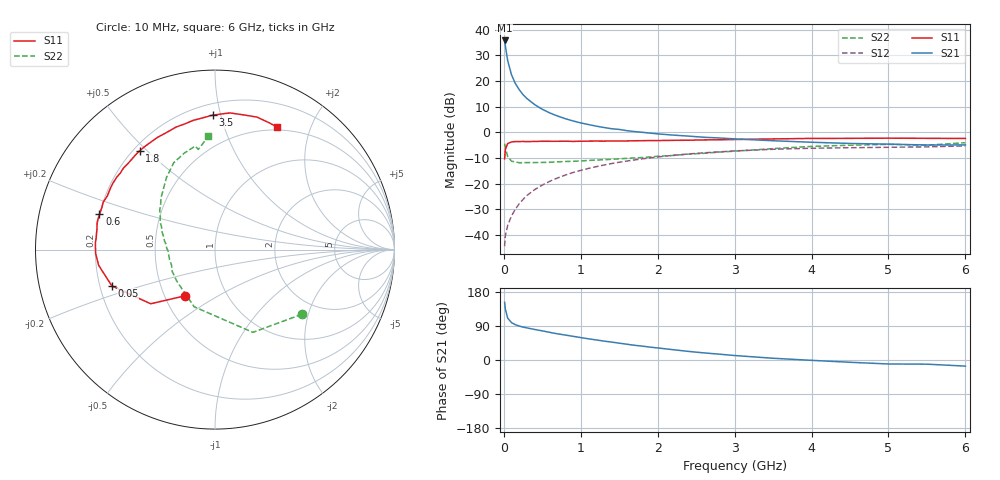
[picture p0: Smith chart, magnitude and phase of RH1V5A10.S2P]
! SIEMENS Small Signal Semiconductors
! BFR106
! Si NPN RF Bipolar Junction Transistor in SOT23
! VCE = 1.5 V  IC = 100 mA
! Common Emitter S-Parameters:  August  1996
# GHz  S  MA  R  50
!  f  S11  S21  S12  S22
! GHz  MAG  ANG  MAG  ANG  MAG  ANG  MAG  ANG
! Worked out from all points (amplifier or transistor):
!   36 points, 10 MHz to 6 GHz, reference 50 ohm
!   highest |S21| = 35.8 dB at 10 MHz (marker M1)
!   |S21| within 3 dB of that: start of sweep to 24.45 MHz
!   unconditionally stable (mu >= 1): 79.45 MHz to end of sweep
!   at 250 MHz: K = 1.24, MAG = 17.5 dB, |S12| = -26.1 dB
!   at 1.4 GHz: K = 1.17, MAG = 4.3 dB, |S12| = -12.1 dB
!   at 6 GHz: K = 1.04, MAG = -1.0 dB, |S12| = -5.2 dB
!   S11 on the Smith chart (normalised r, x): 10 MHz: 0.64, -0.36; 50 MHz: 0.25, -0.16; 600 MHz: 0.20, +0.14; 1.8 GHz: 0.22, +0.48; 3.5 GHz: 0.28, +0.94; 6 GHz: 0.46, +1.52
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0.01  0.306 -122.8  61.98 152.1  0.0061 66.7  0.6041 -36.6
0.02  0.4686 -139.9  48.37 133.8  0.0098 58.6  0.507 -65.4
0.05  0.6093 -160.6  25.07 110.5  0.0155 55.4  0.3389 -110.1
0.1  0.6541 -172.3  13.25 98.6  0.0238 62.6  0.2759 -140.7
0.15  0.6654 -178.2  8.981 93.1  0.032 67.7  0.2677 -153.2
0.2  0.6659 179.1  6.815 89.7  0.041 70.1  0.2574 -160.0
0.25  0.6676 176.6  5.44 86.8  0.0497 71.4  0.2579 -165.6
0.3  0.6652 174.4  4.585 84.7  0.0593 72.2  0.2592 -168.2
0.4  0.668 169.9  3.494 80.6  0.077 72.7  0.2597 -173.2
0.5  0.674 167.0  2.828 76.9  0.0945 72.1  0.2606 -176.8
0.6  0.6732 163.0  2.392 72.8  0.1126 71.1  0.2627 -179.1
0.7  0.6722 159.8  2.086 69.0  0.1302 69.5  0.268 178.8
0.8  0.6765 157.0  1.855 65.8  0.1481 67.9  0.272 176.1
1.1  0.6784 147.1  1.426 55.9  0.1995 62.7  0.2852 170.4
1.4  0.6831 138.2  1.184 47.3  0.2479 57.2  0.3003 164.4
1.8  0.6925 127.2  1.008 36.6  0.3063 49.7  0.3244 156.7
2.2  0.7024 117.3  0.889 27.2  0.3585 42.3  0.3568 148.6
2.6  0.7163 107.6  0.807 18.8  0.4012 35.1  0.3926 140.5
3.5  0.7491 91.0  0.69 4.6  0.4708 20.3  0.4845 123.9
4.5  0.7677 77.5  0.611 -6.0  0.5042 6.3  0.5644 107.6
5.5  0.7684 67.1  0.57 -11.0  0.5239 -1.7  0.566 99.5
6  0.7658 63.3  0.572 -16.1  0.5472 -8.2  0.6313 93.3
